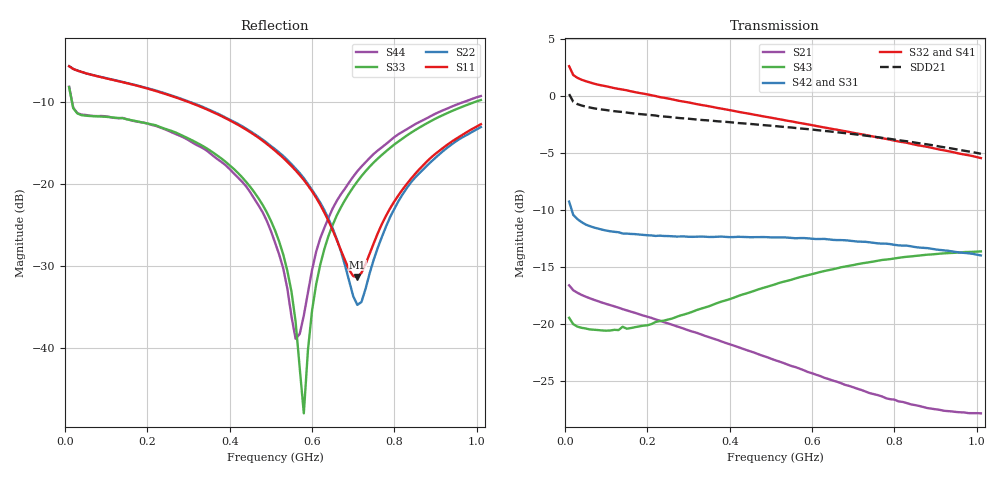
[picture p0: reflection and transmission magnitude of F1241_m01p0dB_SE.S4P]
! Integrated Device Technology
! Corporate Headquarters
! 6024 Silver Creek Valley Road
! San Jose, CA 95138  USA
! Phone:  1-408-284-8200
! Toll Free:  1-800-223-1366
! Webpage:  http://www.idt.com/
! Timing and RF Division
! 515 Groton Road, Suite 102
! Westford, MA 01886-6024
! Device:  F1241
! Description: Dual Intermediate Frequency Digital Variable Gain Amplifier
! Frequency:  10.0 -  500.00 MHz
! Package:  5x5 mm QFN Plastic Package: 32 pin
! Ports:  8 RF, 20 DC
!  Pin  1  = GA3  Pin 17  = RF OUT_B+
!  Pin  2  = GA4  Pin 18  = RF OUT_B-
!  Pin  3  = GA5  Pin 19  = STBY_B
!  Pin  4  = ISET_A  Pin 20  = Ground
!  Pin  5  = ISET_B  Pin 21  = Ground
!  Pin  6  = GB5  Pin 22  = STB_A
!  Pin  7  = GB4  Pin 23  = RF OUT_A-  = Port 4
!  Pin  8  = GB3  Pin 24  = RF OUT_A+  = Port 3
!  Pin  9  = GB2  Pin 25  = NO CONNECT
!  Pin 10  = GB1  Pin 26  = NO CONNECT
!  Pin 11  = RF IN_B+  Pin 27  = VCC
!  Pin 12  = RF IN_B-  Pin 28  = Ground
!  Pin 13  = Ground  Pin 29  = RF IN_A-  = Port 2
!  Pin 14  = VCC  Pin 30  = RF IN_A+  = Port 1
!  Pin 15  = NO CONNECT  Pin 31  = GA1
!  Pin 16  = NO CONNECT  Pin 32  = GA2
! State:  21
! Gain State:  -1.0 dB
! Voltages:  Vcc = +5.00 Volts  Icc approximately 160.0 mA or 80 mA per channel.
! Data:  The device was measured on a custom evaluation board which has
!  individual transmission lines to the RF pins.  Data was collected
!  using a calibrated network analyzer.  The evaluation board was
!  de-embedded using a port reference technique.
!  The reference plane is the edge of the package pin.
!  Only Channel A was measured.
!  This data is in single-ended operation.  If your needs are balanced
!  or differential S-parameters then this file needs to be used a
!  linear simulator.
! Misc:  Lot Code  160028MY
!  Action Tracker AT004
! Date Measured:  2014-08-14
! Date:  2014-08-28  MJV
! Note:
!  Integrated Device Technology supplies this data as a sample of measured
!  data at the package pin for this product.  Your particular data for this
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# Hz S dB R 50
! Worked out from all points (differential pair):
!   101 points, 10 MHz to 1.01 GHz, reference 50 ohm
!   strongest paths, dB at 10 MHz, 260 MHz, 510 MHz, 760 MHz, 1.01 GHz:
!     S32: 2.6, -0.3, -2.0, -3.7, -5.5
!     S41: 2.6, -0.3, -2.1, -3.8, -5.7
!     S42: -9.3, -12.3, -12.4, -12.9, -14.0
!     S31: -9.3, -12.3, -12.5, -13.1, -14.1
!     S43: -19.5, -19.5, -16.5, -14.5, -13.7
!     S21: -16.6, -20.1, -23.2, -26.2, -27.8
!   taken as a pair (ports 2,1 in; 3,4 out), SDD21 dB: 0.1, -1.9, -2.7, -3.7, -5.1
!   lowest |S11| = -31.4 dB at 710 MHz (marker M1), VSWR 1.06, Z = 48 - j1.68 ohm
!   |S11| at or under -10 dB: 299.1 MHz to end of sweep
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1e7  -5.66 -8.9  -16.62 -13.0  -35.32 -1.2  -22.28 9.4
     -16.63 -13.0  -5.65 -8.8  -22.30 9.0  -35.39 -1.2
     -9.28 157.9  2.58 169.7  -8.22 -37.8  -19.53 -178.2
     2.62 169.7  -9.29 158.0  -19.47 -178.3  -8.16 -37.6
4.6e8  -14.03 -40.5  -22.50 -37.1  -34.22 11.7  -23.21 -24.9
       -22.52 -37.6  -13.91 -36.6  -23.06 -24.6  -34.17 10.0
       -12.47 48.7  -1.68 113.0  -21.05 -31.1  -17.24 99.3
       -1.74 111.8  -12.40 48.0  -17.10 99.0  -21.85 -23.8
5.4e8  -17.33 -48.1  -23.48 -38.4  -33.45 10.5  -23.23 -29.5
       -23.56 -38.9  -17.09 -42.7  -22.96 -29.2  -33.44 8.5
       -12.54 33.8  -2.20 104.2  -30.62 -40.1  -16.39 88.0
       -2.30 102.8  -12.44 32.6  -16.23 87.5  -32.80 -8.8
5.8e8  -19.53 -53.2  -23.96 -38.4  -33.06 9.4  -23.23 -31.9
       -24.07 -39.0  -19.32 -46.3  -22.93 -31.5  -33.07 7.4
       -12.60 26.8  -2.46 99.8  -48.00 -141.2  -16.01 82.4
       -2.58 98.5  -12.48 25.7  -15.82 82.0  -36.07 96.3
6.2e8  -22.57 -60.9  -24.45 -38.2  -32.71 8.7  -23.24 -34.3
       -24.58 -38.9  -22.31 -52.1  -22.91 -33.9  -32.66 6.2
       -12.68 20.2  -2.73 95.6  -29.85 148.7  -15.63 77.0
       -2.85 94.2  -12.57 19.0  -15.46 76.8  -26.63 125.1
7.1e8  -31.38 -139.6  -25.52 -36.5  -31.90 5.4  -23.34 -39.7
       -25.68 -36.8  -34.78 -125.2  -22.88 -39.5  -31.90 2.7
       -12.90 6.4  -3.33 86.2  -19.71 139.8  -14.97 65.2
       -3.49 84.8  -12.79 4.6  -14.77 65.1  -18.46 130.4
1.01e9  -12.73 130.7  -27.72 -20.1  -29.92 -9.8  -24.09 -57.5
        -27.84 -18.8  -13.08 130.9  -23.35 -58.2  -29.85 -13.0
        -14.13 -29.9  -5.48 57.5  -9.78 125.4  -13.85 31.3
        -5.73 56.5  -14.00 -33.2  -13.65 31.1  -9.29 121.5
